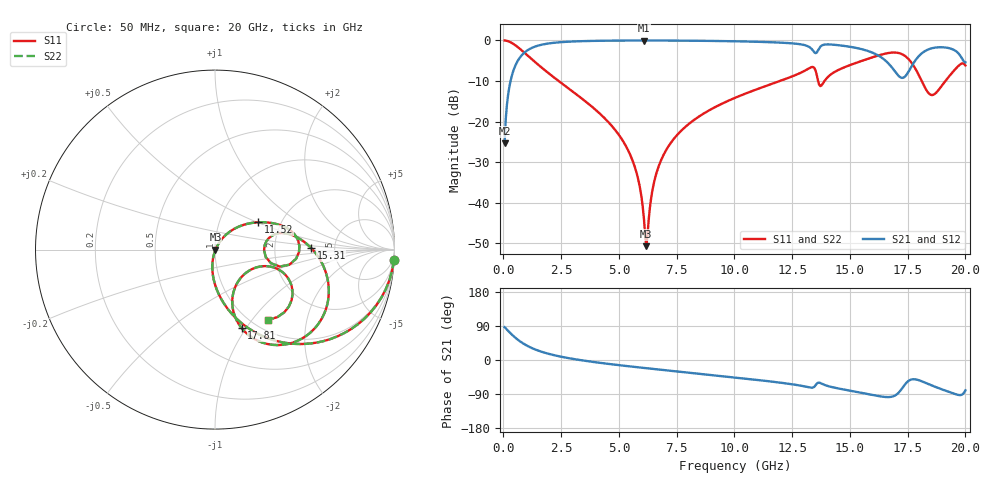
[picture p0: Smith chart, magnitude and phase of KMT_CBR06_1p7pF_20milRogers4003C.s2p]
! Data measured by Modelithics Inc. support@modelithics.com 813-866-6335
! KEMET CBR0603 1.7pF, Pad Width= 0.851mm, Pad Length= 0.64mm, Pad Gap= 0.62mm, 20mil Rogers 4003C substrate Data, January 2022
# hz S ma R 50
! 2 Port Network Data from SP1.SP block
! freq  magS11  angS11  magS21  angS21  magS12  angS12  magS22  angS22
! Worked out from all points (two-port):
!   401 points, 50 MHz to 20 GHz, reference 50 ohm
!   highest |S21| = -0.03 dB at 6.085 GHz (marker M1); lowest = -25.3 dB at 50 MHz (marker M2)
!   |S21| within 3 dB of the highest: 903.7 MHz to 13.48 GHz (12.58 GHz wide, 175 % of centre); 13.55 GHz to 15.98 GHz (2.429 GHz wide, 16.5 % of centre)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
!   lowest |S11| = -50.7 dB at 6.185 GHz (marker M3), VSWR 1.01, Z = 50.3 - j0.119 ohm
!   |S11| at or under -10 dB: 2.389 GHz to 11.97 GHz (9.58 GHz wide, 133 % of centre); 13.62 GHz to 13.9 GHz (278.1 MHz wide, 2.02 % of centre); 18.11 GHz to 19.14 GHz (1.028 GHz wide, 5.52 % of centre)
!   |S22| runs from -50.7 to 0.0 dB; largest |S21 - S12| = 0
!   S11 on the Smith chart (normalised r, x): 50 MHz: 1, -35; 11.52 GHz: 1.53, +0.51; 15.31 GHz: 3.29, +0.10; 17.81 GHz: 0.86, -0.96; 20 GHz: 1.17, -1.21
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5e7  0.9985 -3.3  0.05411 86.7  0.05411 86.7  0.9985 -3.3
3.4925e8  0.9347 -22.0  0.3547 67.9  0.3547 67.9  0.9347 -22.0
7.98125e8  0.7508 -44.1  0.6592 45.9  0.6592 45.9  0.7508 -44.1
1.74575e9  0.4398 -69.8  0.8962 19.9  0.8962 19.9  0.4398 -69.8
3.391625e9  0.1924 -90.1  0.9789 -0.8  0.9789 -0.8  0.1924 -90.1
5.386625e9  0.04487 -102.8  0.9961 -16.3  0.9961 -16.3  0.04487 -102.8
5.8355e9  0.01935 -100.9  0.9968 -19.3  0.9968 -19.3  0.01935 -100.9
6.084875e9  0.006201 -83.2  0.9969 -21.0  0.9969 -21.0  0.006201 -83.2
6.184625e9  0.002914 -24.1  0.9969 -21.6  0.9969 -21.6  0.002914 -24.1
6.73325e9  0.02876 58.8  0.9963 -25.2  0.9963 -25.2  0.02876 58.8
7.8305e9  0.0838 55.6  0.9928 -32.1  0.9928 -32.1  0.0838 55.6
1.0025e10  0.196 42.6  0.9757 -46.0  0.9757 -46.0  0.196 42.6
1.152125e10  0.2848 32.3  0.9512 -56.3  0.9512 -56.3  0.2848 32.3
1.336662e10  0.4706 2.5  0.7716 -73.0  0.7716 -73.0  0.4706 2.5
1.376562e10  0.2781 5.2  0.8582 -62.0  0.8582 -62.0  0.2781 5.2
1.531175e10  0.5342 1.1  0.8038 -84.4  0.8038 -84.4  0.5342 1.1
1.670825e10  0.7019 -28.5  0.505 -97.7  0.505 -97.7  0.7019 -28.5
1.725688e10  0.6762 -50.0  0.345 -75.1  0.345 -75.1  0.6762 -50.0
1.78055e10  0.4632 -71.2  0.552 -50.9  0.552 -50.9  0.4632 -71.2
1.855362e10  0.2123 -44.0  0.8009 -67.4  0.8009 -67.4  0.2123 -44.0
1.935162e10  0.3772 -17.6  0.7944 -85.5  0.7944 -85.5  0.3772 -17.6
2e10  0.491 -52.7  0.5376 -80.2  0.5376 -80.2  0.491 -52.7
